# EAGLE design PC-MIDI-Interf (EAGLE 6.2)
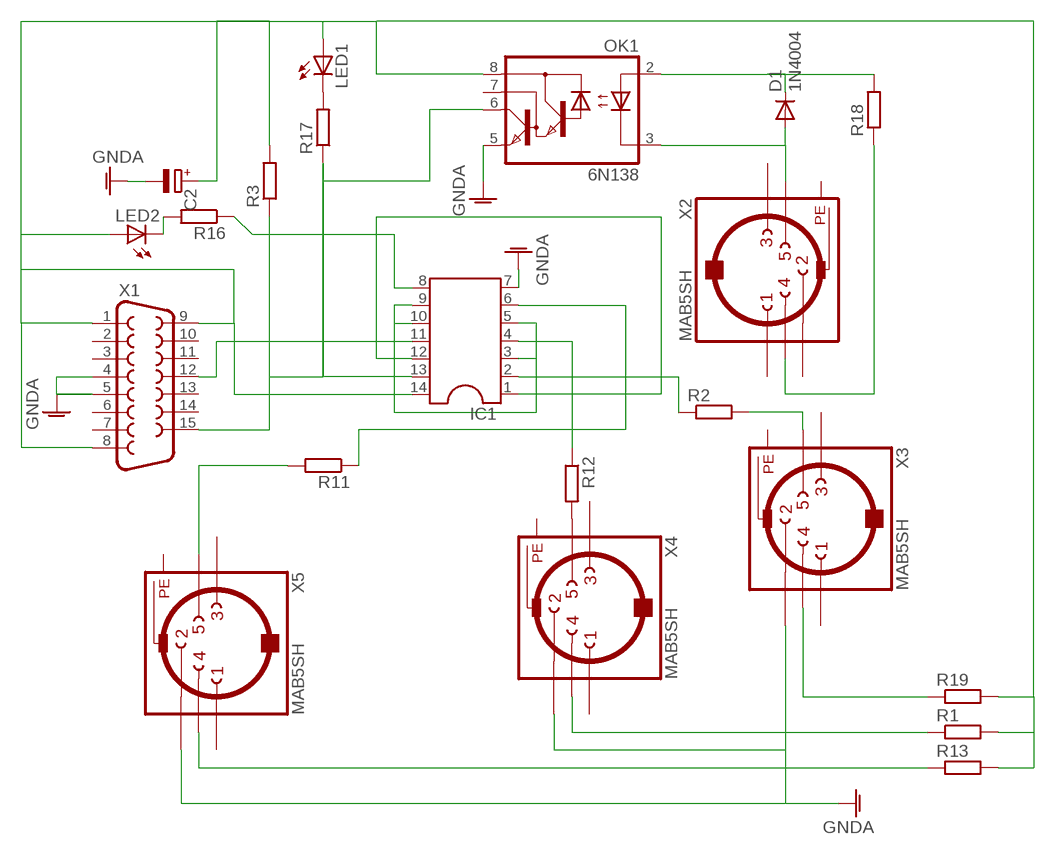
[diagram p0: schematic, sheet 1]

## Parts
C2  CPOL-EUE2-4  [E2-4]
D1  1N4004  [DO41-10]
IC1  DIL14  [DIL14]
LED1  LED3MM  [LED3MM]
LED2  LED3MM  [LED3MM]
OK1  6N138  [DIL08]
R1  R-EU_0204/5  [0204/5]
R2  R-EU_0204/5  [0204/5]
R3  R-EU_0204/5  [0204/5]
R11  R-EU_0204/5  [0204/5]
R12  R-EU_0204/5  [0204/5]
R13  R-EU_0204/5  [0204/5]
R16  R-EU_0204/5  [0204/5]
R17  R-EU_0204/5  [0204/5]
R18  R-EU_0204/5  [0204/5]
R19  R-EU_0204/5  [0204/5]
X1  F15H  [F15H]
X2  MAB5SH  [MAB5SH]
X3  MAB5SH  [MAB5SH]
X4  MAB5SH  [MAB5SH]
X5  MAB5SH  [MAB5SH]

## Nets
GNDA: C2.- IC1.7 OK1.5(GND) X1.4 X1.5 X3.2 X4.2 X5.2
N$1: D1.C OK1.2(A) R18.2
N$2: D1.A OK1.3(C) X2.5
N$3: R11.2 X5.5
N$4: C2.+ IC1.14 LED1.A LED2.A OK1.8(VCC) R1.2 R3.2 R13.2 R19.2 X1.1 X1.8 X1.9
N$5: R19.1 X3.4
N$6: R1.1 X4.4
N$7: R13.1 X5.4
N$8: R12.2 X4.5
N$9: R18.1 X2.4
N$10: R2.2 X3.5
N$11: LED1.K(C) R17.2
N$13: IC1.11 X1.12
N$14: IC1.8 R16.1
N$15: IC1.1 IC1.12
N$16: IC1.13 OK1.6(VO) R3.1 R17.1 X1.15
N$17: LED2.K(C) R16.2
N$19: IC1.6 R11.1
N$20: IC1.4 R12.1
N$21: IC1.2 R2.1
N$23: IC1.3 IC1.5 IC1.9 IC1.10
Unconnected: OK1.7(VB) X1.2 X1.3 X1.6 X1.7 X1.10 X1.11 X1.13 X1.14 X2.1 X2.2 X2.3 X3.1 X3.3 X4.1 X4.3 X5.1 X5.3

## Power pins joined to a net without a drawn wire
PE: X2.PE X2.PE@(PE) X3.PE X3.PE@(PE) X4.PE X4.PE@(PE) X5.PE X5.PE@(PE)

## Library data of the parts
C2 = rcl:CPOL-EU: POLARIZED CAPACITOR, European symbol
D1 = diode:1N4004: DIODE
IC1 = ic-package:DIL14: Dual In Line / Socket
LED1 LED2 = led:LED: LED
OK1 = optocoupler:6N138: MOTOROLA OPTO COUPLER; MF: VISHAY/TELEFUNKEN; MPN: 6N138; OC_FARNELL: 9860150; OC_NEWARK: 35K5294
R1-R3 R11-R13 R16-R19 = rcl:R-EU_: RESISTOR, European symbol
X1 = con-subd:F15: SUB-D; OC_FARNELL: unknown; OC_NEWARK: unknown
X2-X5 = con-hirschmann:MAB5SH: Female CONNECTOR 5 pins 90 deg. with shield, horizontal (DIN 41524); OC_FARNELL: 809883; OC_NEWARK: unknown

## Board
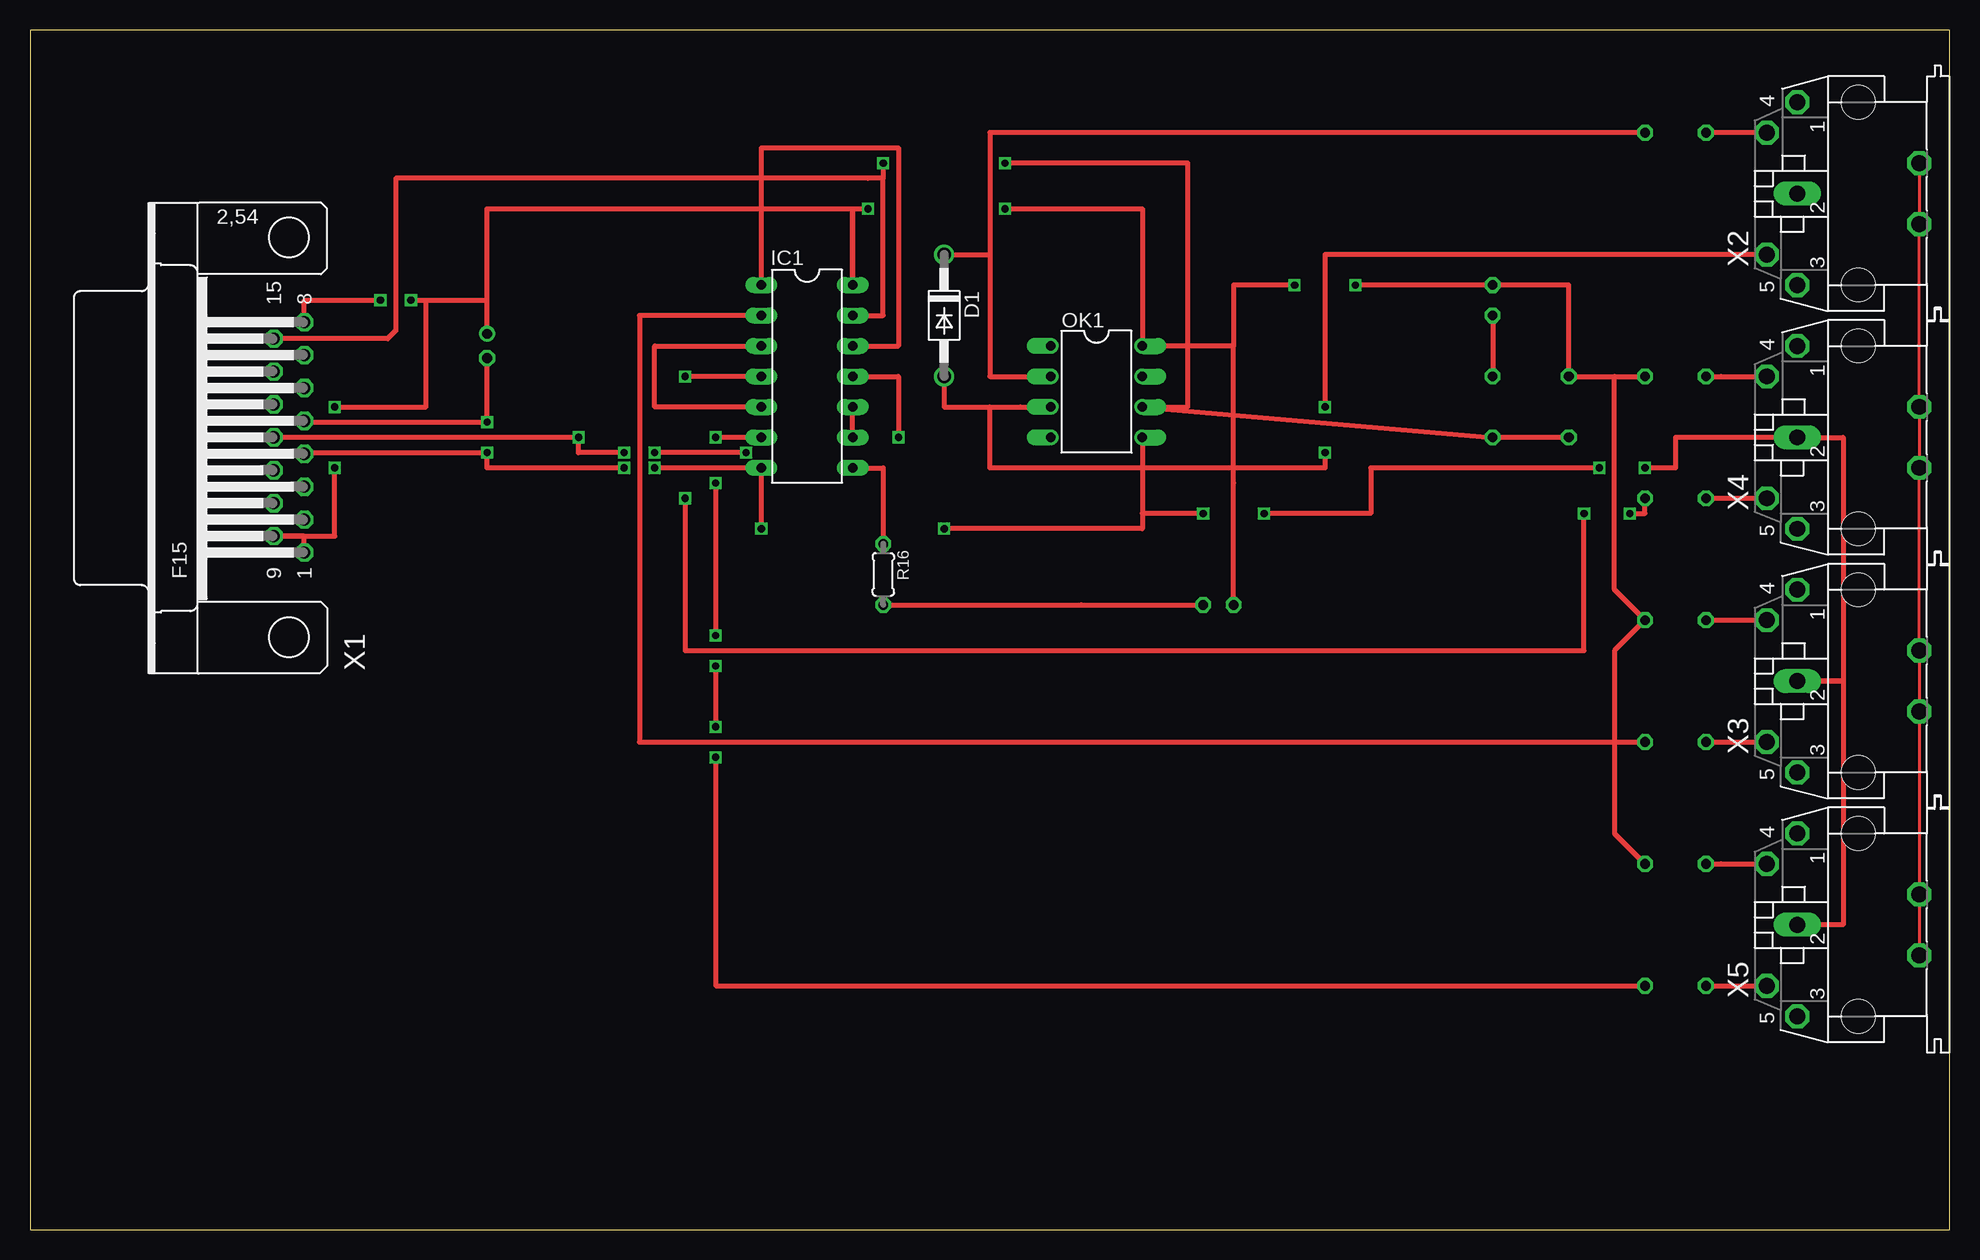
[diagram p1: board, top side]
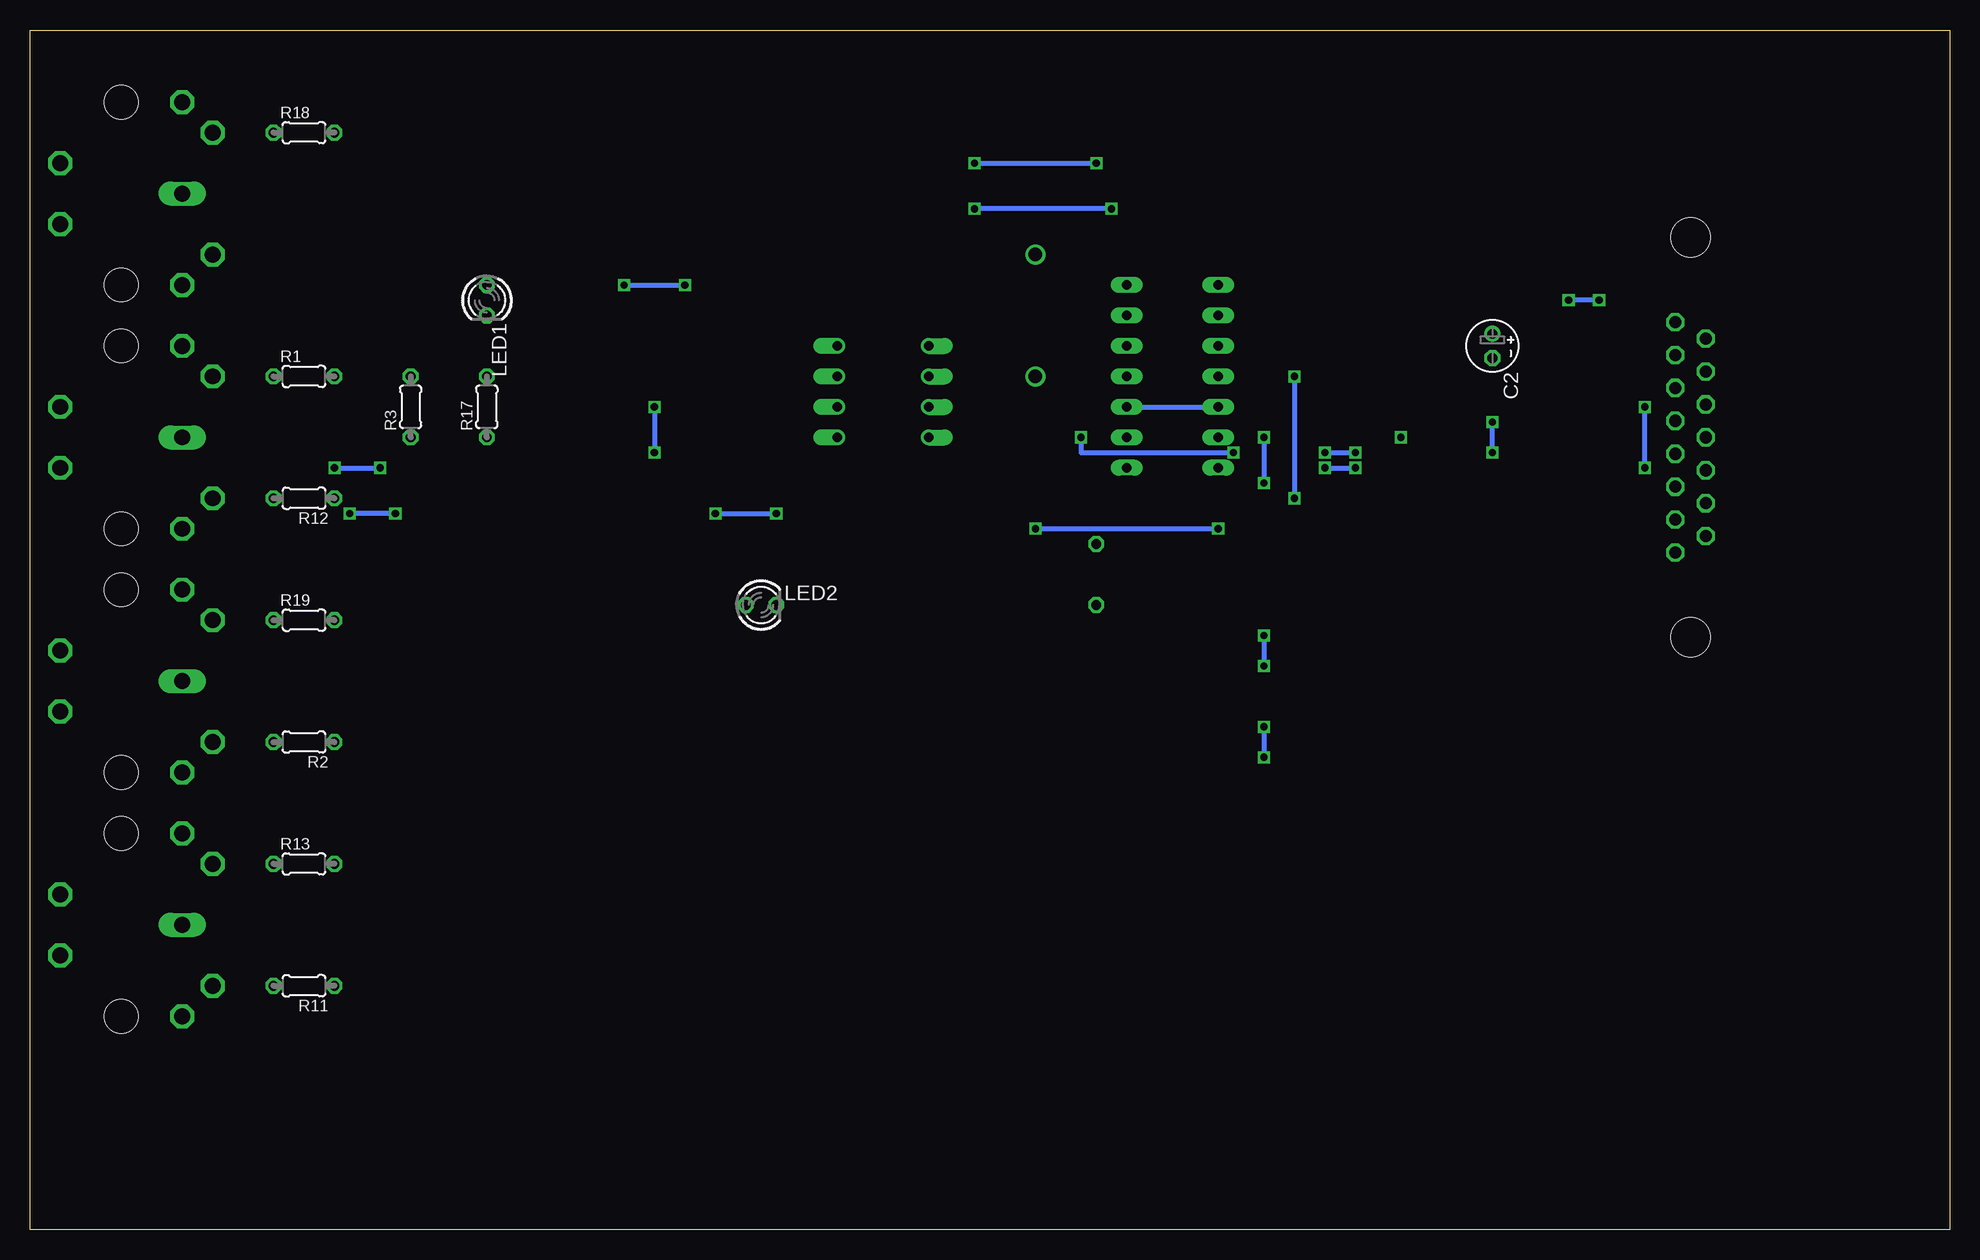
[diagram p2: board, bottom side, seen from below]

Size 160 x 100 mm. Coordinates in mm from the lower left corner, seen from the top.
Outline: 0,0 160,0 160,100 0,100 0,0
Copper layers (1*16): Top 0.035mm / dielectric 1.5mm / Bottom 0.035mm
Design rules: minimum track width 10mil, minimum drill 24mil, track to track 8mil, track to pad 8mil, pad to pad 8mil, via to via 8mil, smd to smd 8mil, copper to edge 40mil, drill to drill 8mil, minimum pad ring 10mil, minimum via ring 8mil, stop-mask expansion 4mil, vias tented up to drill 0mil, thermal gap 10mil

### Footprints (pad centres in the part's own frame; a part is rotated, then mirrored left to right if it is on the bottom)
E2-4 = drill 0.813 pad 1.27: + -1.016,0 | drill 0.813 pad 1.27 octagon: - 1.016,0
DO41-10 = drill 1.118: A 5.08,0; C -5.08,0
DIL14 = drill 0.813 long: 1 -7.62,-3.81; 2 -5.08,-3.81; 3 -2.54,-3.81; 4 0,-3.81; 5 2.54,-3.81; 6 5.08,-3.81; 7 7.62,-3.81; 8 7.62,3.81; 9 5.08,3.81; 10 2.54,3.81; 11 0,3.81; 12 -2.54,3.81; 13 -5.08,3.81; 14 -7.62,3.81
LED3MM = drill 0.813 octagon: A -1.27,0; K 1.27,0
DIL08 = drill 0.813 offset: 1 -3.81,-3.81; 2 -1.27,-3.81; 3 1.27,-3.81; 4 3.81,-3.81; 5 3.81,3.81; 6 1.27,3.81; 7 -1.27,3.81; 8 -3.81,3.81
0204/5 = drill 0.813 octagon: 1 -2.54,0; 2 2.54,0
F15H = drill 1.016 octagon: 1 -9.601,-1.27; 2 -6.858,-1.27; 3 -4.115,-1.27; 4 -1.372,-1.27; 5 1.372,-1.27; 6 4.115,-1.27; 7 6.858,-1.27; 8 9.601,-1.27; 9 -8.23,1.27; 10 -5.486,1.27; 11 -2.743,1.27; 12 0,1.27; 13 2.743,1.27; 14 5.486,1.27; 15 8.23,1.27 | hole 3.302: -16.662,0; 16.662,0
MAB5SH = drill 1.321 octagon: 1 7.62,5.08; 3 -7.62,5.08; 4 5.08,7.62; 5 -5.08,7.62; PE -2.54,-5.08; PE@ 2.54,-5.08 | drill 1.321 long: 2 0,5.08 | hole 2.794: 7.62,0; -7.62,0

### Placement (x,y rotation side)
C2  38.1,73.66 270 bottom
D1  76.2,76.2 270 top
IC1  64.77,71.12 270 top
LED1  121.92,77.47 270 bottom
LED2  99.06,52.07 0 bottom
OK1  88.9,69.85 270 top
R1  137.16,71.12 0 bottom
R2  137.16,40.64 180 bottom
R3  128.27,68.58 90 bottom
R11  137.16,20.32 180 bottom
R12  137.16,60.96 180 bottom
R13  137.16,30.48 0 bottom
R16  71.12,54.61 270 top
R17  121.92,68.58 90 bottom
R18  137.16,91.44 0 bottom
R19  137.16,50.8 0 bottom
X1  21.59,66.04 90 top
X2  152.4,86.36 90 top
X3  152.4,45.72 90 top
X4  152.4,66.04 90 top
X5  152.4,25.4 90 top

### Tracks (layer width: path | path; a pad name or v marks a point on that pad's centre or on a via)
GNDA  (via drill 0.6)
  Top 0.406: OK1.5 92.71,59.69 | 92.71,59.69 92.71,58.42 v76.2,58.42 | v60.96,58.42 IC1.7 v52.07,63.5 | C2.- v38.1,67.31 22.86,67.31 X1.5 | 151.13,45.72 151.13,66.04 X4.2 137.16,66.04 137.16,63.5 v134.62,63.5 | 151.13,45.72 X3.2 151.13,45.72 | 151.13,45.72 151.13,25.4 X5.2 | v130.81,63.5 111.76,63.5 111.76,59.69 v102.87,59.69 | v97.79,59.69 92.71,59.69 | v22.86,64.77 v38.1,64.77 38.1,63.5 v49.53,63.5
  Bottom 0.406: v76.2,58.42 v60.96,58.42 | X1.4 v22.86,64.77 | v134.62,63.5 v130.81,63.5 | v102.87,59.69 v97.79,59.69 | v38.1,64.77 v38.1,67.31 | v52.07,63.5 v49.53,63.5
N$1
  Top 0.406: D1.C 80.01,81.28 | 80.01,81.28 80.01,71.12 OK1.2 | R18.2 80.01,91.44 80.01,81.28
N$2  (via drill 0.6)
  Top 0.406: D1.A 76.2,68.58 80.01,68.58 | 80.01,68.58 82.55,68.58 OK1.3 | X2.5 107.95,81.28 v107.95,68.58 | v107.95,64.77 107.95,63.5 102.87,63.5 80.01,63.5 80.01,68.58
  Bottom 0.406: v107.95,68.58 v107.95,64.77
N$3
  Top 0.406: R11.2 X5.5
N$4  (via drill 0.6)
  Top 0.406: C2.+ 38.1,77.47 | 38.1,77.47 38.1,85.09 68.58,85.09 | 68.58,85.09 IC1.14 68.58,85.09 | 132.08,71.12 R3.2 128.27,78.74 LED1.A v110.49,78.74 | 132.08,71.12 R1.2 | 132.08,71.12 132.08,53.34 R19.2 132.08,48.26 132.08,34.29 132.08,33.02 R13.2 | LED2.A 100.33,62.23 100.33,73.66 | 100.33,73.66 96.52,73.66 | 96.52,73.66 OK1.8 92.71,85.09 v81.28,85.09 | X1.1 22.86,57.81 X1.9 25.4,57.81 v25.4,63.5 | 22.86,77.47 X1.8 22.86,77.47 | 22.86,77.47 v29.21,77.47 | v31.75,77.47 33.02,77.47 | 33.02,77.47 38.1,77.47 | v105.41,78.74 100.33,78.74 100.33,73.66 | 100.33,73.66 96.52,73.66 | 68.58,85.09 v69.85,85.09 | v25.4,68.58 33.02,68.58 33.02,77.47
  Bottom 0.406: v29.21,77.47 v31.75,77.47 | v110.49,78.74 v105.41,78.74 | v69.85,85.09 v81.28,85.09 | v25.4,63.5 v25.4,68.58
N$5
  Top 0.406: R19.1 X3.4
N$6
  Top 0.406: R1.1 140.97,71.12 X4.4
N$7
  Top 0.406: R13.1 140.97,30.48 X5.4
N$8
  Top 0.406: R12.2 X4.5
N$9
  Top 0.406: X2.4 R18.1
N$10
  Top 0.406: R2.2 X3.5
N$11
  Top 0.406: LED1.K R17.2
N$13  (via drill 0.6)
  Top 0.406: 72.39,71.12 IC1.11 72.39,71.12 | 72.39,71.12 v72.39,66.04 72.39,71.12 | X1.12 v45.72,66.04 45.72,64.77 v49.53,64.77 | v59.69,64.77 v52.07,64.77
  Bottom 0.406: v72.39,66.04 72.39,64.77 v59.69,64.77 | v52.07,64.77 v49.53,64.77
N$14
  Top 0.406: IC1.8 71.12,63.5 R16.1
N$15
  Top 0.406: IC1.12 72.39,73.66 72.39,90.17 63.5,90.17 60.96,90.17 IC1.1
N$16  (via drill 0.6)
  Top 0.406: IC1.13 71.12,76.2 71.12,87.63 | 71.12,87.63 69.85,87.63 30.48,87.63 30.48,74.93 29.82,74.27 X1.15 | R3.1 R17.1 OK1.6 96.52,68.58 96.52,88.9 v81.28,88.9 | v71.12,88.9 71.12,87.63
  Bottom 0.406: v81.28,88.9 v71.12,88.9
N$17
  Top 0.406: R16.2 87.63,52.07 LED2.K
N$19  (via drill 0.6)
  Top 0.406: IC1.6 v57.15,66.04 | v57.15,62.23 v57.15,49.53 | v57.15,46.99 v57.15,41.91 | v57.15,39.37 57.15,20.32 R11.1
  Bottom 0.406: v57.15,66.04 v57.15,62.23 | v57.15,49.53 v57.15,46.99 | v57.15,41.91 v57.15,39.37
N$20  (via drill 0.6)
  Top 0.406: IC1.4 v54.61,71.12 | v54.61,60.96 54.61,48.26 129.54,48.26 v129.54,59.69 | v133.35,59.69 134.62,59.69 R12.1
  Bottom 0.406: v54.61,71.12 v54.61,60.96 | v129.54,59.69 v133.35,59.69
N$21
  Top 0.406: IC1.2 50.8,76.2 50.8,40.64 R2.1
N$23
  Top 0.406: IC1.5 52.07,68.58 52.07,73.66 IC1.3 | IC1.9 IC1.10
  Bottom 0.406: IC1.10 IC1.5
PE
  Top 0.254: X2.PE@ X2.PE X4.PE@ X4.PE X3.PE@ X3.PE X5.PE@ X5.PE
